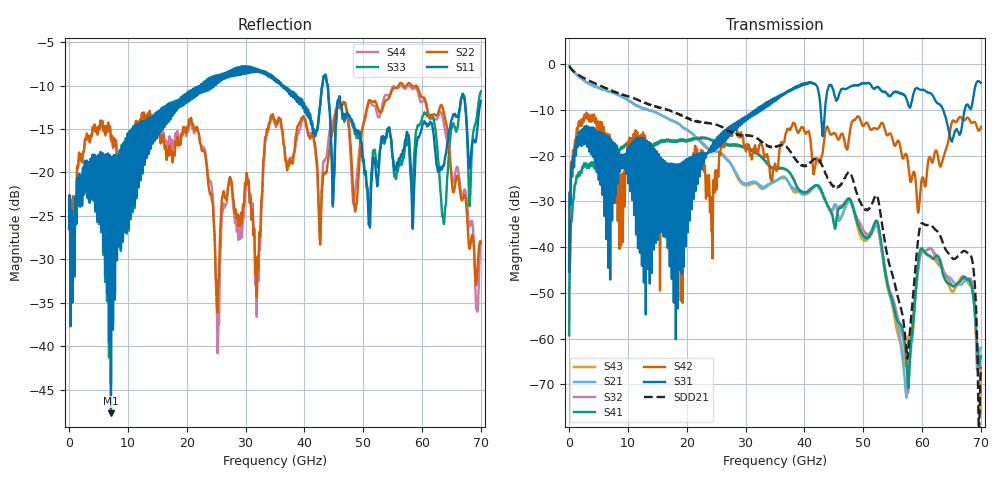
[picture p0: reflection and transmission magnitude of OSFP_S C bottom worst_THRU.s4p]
! AWR Design Environment (8415) Mon Jan 07 17:50:58 2019
! Document = 'OSFP Channel_S'
! nPorts: 4, nXvals: 7001
# HZ S DB R 50
!Freq DBS11 AngS11 DBS12 AngS12 DBS13 AngS13 DBS14 AngS14
!	DBS21 AngS21 DBS22 AngS22 DBS23 AngS23 DBS24 AngS24
!	DBS31 AngS31 DBS32 AngS32 DBS33 AngS33 DBS34 AngS34
!	DBS41 AngS41 DBS42 AngS42 DBS43 AngS43 DBS44 AngS44
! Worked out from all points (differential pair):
!   7000 points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, 10 MHz to 70 GHz, reference 50 ohm
!   strongest paths, dB at 10 MHz, 17.51 GHz, 35.01 GHz, 52.51 GHz, 70 GHz:
!     S31: -45.4, -29.5, -7.4, -4.9, -4.0
!     S42: -45.4, -30.8, -21.7, -14.0, -13.7
!     S41: -59.2, -16.8, -22.9, -34.9, -63.9
!     S32: -59.3, -16.7, -22.9, -35.8, -66.6
!     S21: -0.4, -12.3, -25.6, -36.0, -62.1
!     S43: -0.4, -12.3, -25.7, -35.3, -76.4
!   taken as a pair (ports 1,3 in; 2,4 out), SDD21 dB: -0.4, -10.3, -18.1, -29.4, -66.3
!   lowest |S11| = -47.7 dB at 7.12 GHz (marker M1), VSWR 1.01, Z = 50.1 - j0.408 ohm
!   |S11| at or under -10 dB: start of sweep to 22.43 GHz; 36.33 GHz to 43.05 GHz (6.718 GHz wide, 16.9 % of centre); 43.97 GHz to end of sweep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
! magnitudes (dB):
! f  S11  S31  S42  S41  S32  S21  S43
! 10 MHz  -26.5  -45.4  -45.4  -59.2  -59.3  -0.4  -0.4
! 7.12 GHz  -47.7  -16.7  -17.0  -21.1  -21.2  -6.1  -6.1
! 52.28 GHz  -20.8  -5.0  -14.2  -34.2  -34.8  -35.3  -34.5
! 57.3 GHz  -15.9  -7.5  -19.6  -63.8  -65.0  -72.8  -64.0
! 59.97 GHz  -14.9  -5.6  -25.1  -40.3  -41.1  -41.0  -40.4
! 67.26 GHz  -11.6  -9.9  -12.2  -46.6  -47.0  -47.4  -46.5
! 70 GHz  -11.8  -4.0  -13.7  -63.9  -66.6  -62.1  -76.4
